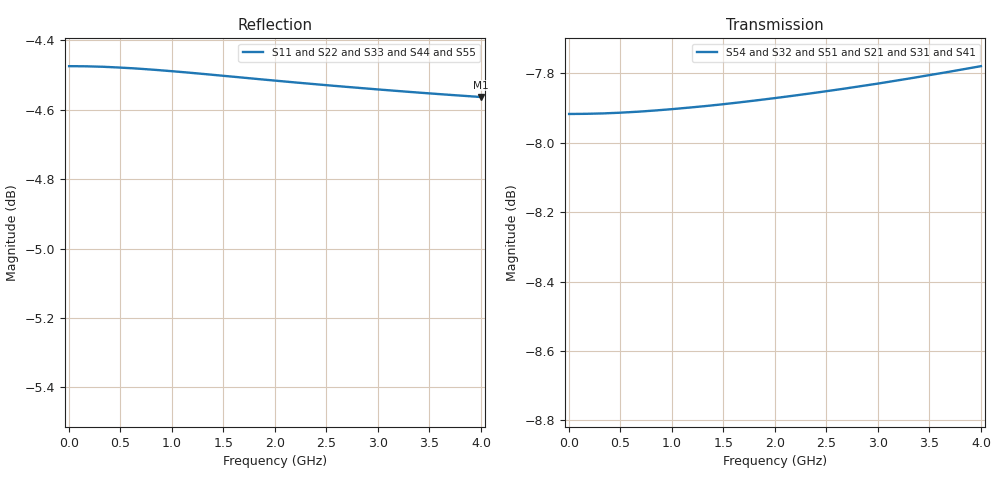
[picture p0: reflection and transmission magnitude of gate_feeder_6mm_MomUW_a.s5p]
! Created Thu Sep 17 15:57:11 2015
# ghz S ma R 50
! 5 Port Network Data from data block
! freq  magS11  angS11  magS12  angS12  magS13  angS13  magS14  angS14
!  magS15  angS15
!  magS21  angS21  magS22  angS22  magS23  angS23
!  magS24  angS24  magS25  angS25
!  magS31  angS31  magS32  angS32
!  magS33  angS33  magS34  angS34  magS35  angS35
!  magS41  angS41
!  magS42  angS42  magS43  angS43  magS44  angS44  magS45  angS45
!  magS51  angS51  magS52  angS52  magS53  angS53  magS54  angS54
!  magS55  angS55
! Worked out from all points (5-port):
!   23 points, 1 MHz to 4 GHz, reference 50 ohm
!   strongest paths, dB at 1 MHz, 500.9 MHz, 1.501 GHz, 2.5 GHz, 4 GHz:
!     S54: -7.9, -7.9, -7.9, -7.9, -7.8
!     S32: -7.9, -7.9, -7.9, -7.9, -7.8
!     S51: -8.0, -8.0, -8.0, -8.0, -8.0
!     S21: -8.0, -8.0, -8.0, -8.0, -8.0
!     S31: -8.0, -8.0, -8.0, -8.0, -8.0
!     S41: -8.0, -8.0, -8.0, -8.0, -8.0
!   lowest |S11| = -4.6 dB at 4 GHz (marker M1), VSWR 3.89, Z = 12.8 + j1.13 ohm
!   |S11| at or under -10 dB: nowhere
